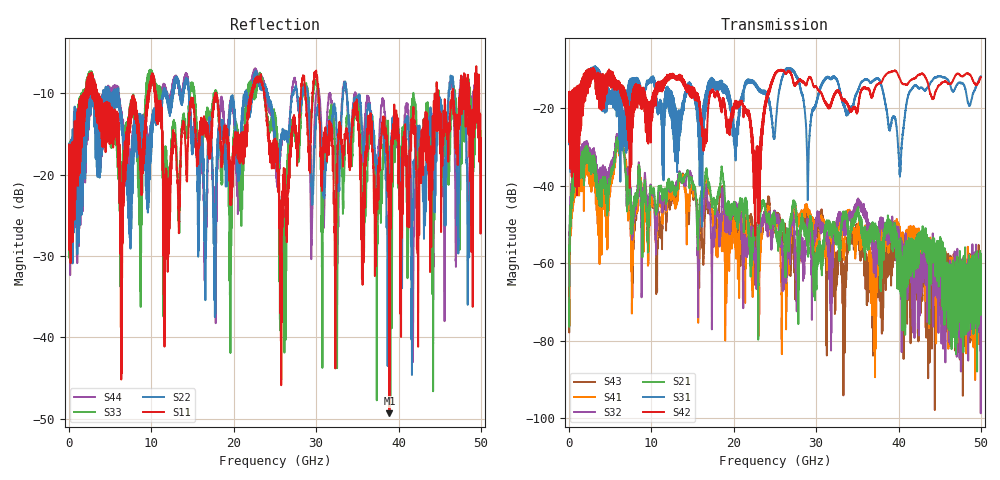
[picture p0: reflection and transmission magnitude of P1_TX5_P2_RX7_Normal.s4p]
!Keysight Technologies,N5225B,MY57041031,A.13.20.10
!Date: Friday, May 31, 2019 11:38:50
!Correction: S11(Full 4 Port(1,2,3,4))
!S12(Full 4 Port(1,2,3,4))
!S13(Full 4 Port(1,2,3,4))
!S14(Full 4 Port(1,2,3,4))
!S21(Full 4 Port(1,2,3,4))
!S22(Full 4 Port(1,2,3,4))
!S23(Full 4 Port(1,2,3,4))
!S24(Full 4 Port(1,2,3,4))
!S31(Full 4 Port(1,2,3,4))
!S32(Full 4 Port(1,2,3,4))
!S33(Full 4 Port(1,2,3,4))
!S34(Full 4 Port(1,2,3,4))
!S41(Full 4 Port(1,2,3,4))
!S42(Full 4 Port(1,2,3,4))
!S43(Full 4 Port(1,2,3,4))
!S44(Full 4 Port(1,2,3,4))
!S4P File: Measurements: <S11,S12,S13,S14>,
!<S21,S22,S23,S24>,
!<S31,S32,S33,S34>,
!<S41,S42,S43,S44>:
# Hz S  dB  R 50.0
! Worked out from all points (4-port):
!   5000 points, 10 MHz to 50 GHz, reference 50 ohm
!   strongest paths, dB at 10 MHz, 12.51 GHz, 25.01 GHz, 37.51 GHz, 50 GHz:
!     S42: -19.3, -12.1, -11.3, -13.7, -11.9
!     S31: -19.3, -23.1, -26.2, -12.3, -11.7
!     S21: -70.6, -40.0, -48.7, -53.8, -60.0
!     S32: -61.1, -39.4, -47.3, -52.6, -61.6
!     S41: -61.9, -42.6, -50.8, -57.6, -68.4
!     S43: -69.4, -43.6, -50.1, -57.4, -69.0
!   lowest |S11| = -49.3 dB at 38.9 GHz (marker M1), VSWR 1.01, Z = 49.7 - j0.114 ohm
!   |S11| at or under -10 dB: 3.501 GHz to 9.606 GHz (6.105 GHz wide, 93.2 % of centre); 10.5 GHz to 17.79 GHz (7.286 GHz wide, 51.5 % of centre); 30.27 GHz to 44.61 GHz (14.34 GHz wide, 38.3 % of centre)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
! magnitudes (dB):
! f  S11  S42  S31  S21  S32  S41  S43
! 10 MHz  -19.7  -19.3  -19.3  -70.6  -61.1  -61.9  -69.4
! 5.94 GHz  -15.7  -14.2  -21.7  -27.8  -27.3  -28.5  -28.2
! 7.73 GHz  -12.2  -16.0  -15.0  -47.1  -48.2  -52.5  -55.3
! 22.8 GHz  -8.0  -36.8  -14.3  -52.1  -62.7  -54.1  -55.2
! 25.28 GHz  -17.8  -10.3  -19.3  -54.3  -48.6  -47.8  -47.6
! 38.9 GHz  -49.3  -10.7  -25.5  -52.1  -52.5  -51.8  -58.0
! 50 GHz  -15.5  -11.9  -11.7  -60.0  -61.6  -68.4  -69.0
